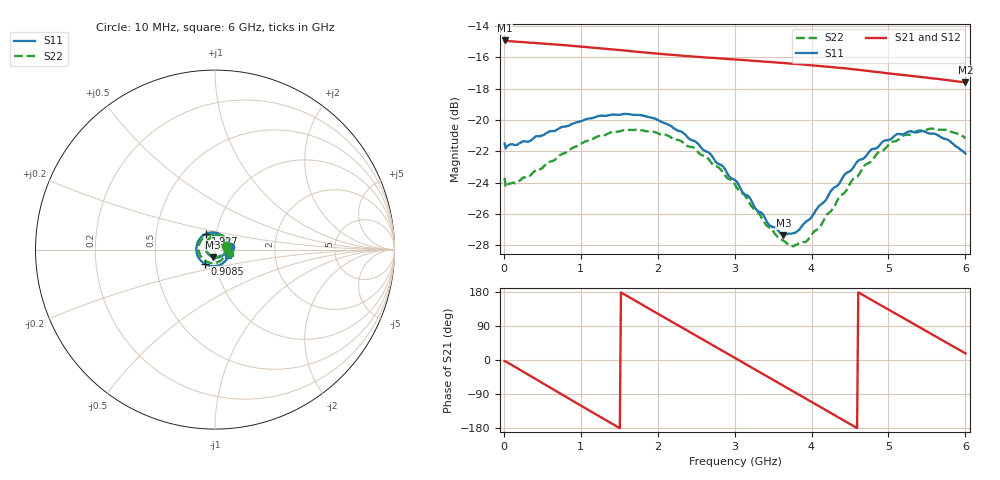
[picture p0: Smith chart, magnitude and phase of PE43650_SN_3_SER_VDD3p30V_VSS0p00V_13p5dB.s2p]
!Keysight Technologies,N5245B,MY57181451,A.13.50.07
!Date: Tuesday, May 07, 2019 08:00:12
!Correction: S11(Full 2 Port(1,2))
!S21(Full 2 Port(1,2))
!S12(Full 2 Port(1,2))
!S22(Full 2 Port(1,2))
!S2P File: Measurements: S11, S21, S12, S22:
# Hz S  dB  R 50
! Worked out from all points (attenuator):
!   401 points, 10 MHz to 6 GHz, reference 50 ohm
!   highest |S21| = -14.94 dB at 10 MHz (marker M1); lowest = -17.6 dB at 6 GHz (marker M2)
!   lowest |S11| = -27.3 dB at 3.634 GHz (marker M3), VSWR 1.09, Z = 48.7 - j4.02 ohm
!   |S11| at or under -10 dB: start of sweep to end of sweep
!   |S22| runs from -28.0 to -20.6 dB; largest |S21 - S12| = 0.0018
!   S11 on the Smith chart (normalised r, x): 10 MHz: 1.18, +0.04; 908.5 MHz: 0.88, -0.14; 1.927 GHz: 0.89, +0.16; 6 GHz: 1.15, -0.07
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1e7  -21.51 10.4  -14.94 -3.4  -15.00 -3.2  -23.69 17.1
2.34625e8  -21.40 -34.9  -15.04 -28.9  -15.10 -28.8  -23.74 -35.0
5.04175e8  -20.99 -72.4  -15.13 -61.2  -15.18 -61.1  -23.05 -73.3
9.085e8  -20.22 -124.7  -15.29 -109.3  -15.34 -109.3  -21.75 -124.1
1.013325e9  -20.07 -137.6  -15.34 -121.7  -15.39 -121.7  -21.50 -136.5
1.462575e9  -19.66 171.0  -15.52 -174.7  -15.59 -174.7  -20.75 174.7
1.6872e9  -19.68 146.2  -15.64 158.9  -15.70 158.9  -20.65 151.3
1.9268e9  -19.86 120.3  -15.74 130.9  -15.79 131.0  -20.73 126.9
2.01665e9  -20.03 110.9  -15.78 120.4  -15.83 120.5  -20.88 117.9
2.241275e9  -20.63 86.5  -15.87 94.2  -15.93 94.3  -21.27 94.7
2.4659e9  -21.34 61.2  -15.97 68.2  -16.02 68.1  -21.77 71.7
2.750425e9  -22.65 29.0  -16.06 35.0  -16.12 35.1  -22.94 40.7
3.005e9  -23.85 -4.0  -16.14 5.4  -16.20 5.5  -24.11 11.5
3.3045e9  -25.81 -48.2  -16.26 -29.5  -16.30 -29.4  -25.91 -29.4
3.63395e9  -27.34 -106.2  -16.37 -67.9  -16.42 -67.9  -27.70 -83.7
3.7837e9  -27.20 -134.7  -16.43 -85.4  -16.48 -85.3  -27.97 -111.5
4.008325e9  -26.14 -174.4  -16.51 -111.6  -16.57 -111.6  -27.27 -152.7
4.517475e9  -23.21 115.2  -16.76 -171.0  -16.82 -170.9  -23.91 132.5
4.757075e9  -21.97 88.1  -16.89 161.1  -16.94 161.2  -22.70 105.6
5.01165e9  -21.27 62.3  -17.03 131.6  -17.09 131.7  -21.52 78.2
5.475875e9  -20.75 19.3  -17.29 77.9  -17.34 78.1  -20.68 33.8
6e9  -22.14 -22.8  -17.60 17.6  -17.65 17.6  -21.16 -11.6
